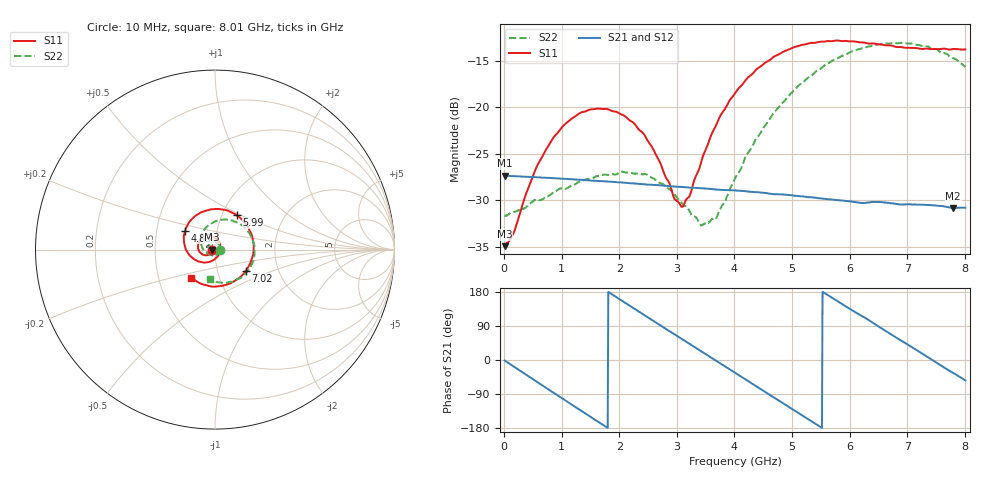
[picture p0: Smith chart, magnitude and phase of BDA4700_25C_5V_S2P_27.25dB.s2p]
!Agilent Technologies,E5071B,MY42404982,A.09.10
!Date: Mon Oct 20 13:40:14 2025
!Data & Calibration Information:
!Freq	S11:SOLT2(ON)	S21:SOLT2(ON)	S12:SOLT2(ON)	S22:SOLT2(ON)
# Hz S RI R 50
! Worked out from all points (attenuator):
!   801 points, 10 MHz to 8.01 GHz, reference 50 ohm
!   highest |S21| = -27.32 dB at 10 MHz (marker M1); lowest = -30.8 dB at 7.8 GHz (marker M2)
!   lowest |S11| = -34.9 dB at 10 MHz (marker M3), VSWR 1.04, Z = 48.2 - j0.0925 ohm
!   |S11| at or under -10 dB: start of sweep to end of sweep
!   |S22| runs from -32.7 to -13.0 dB; largest |S21 - S12| = 0.00037
!   S11 on the Smith chart (normalised r, x): 10 MHz: 0.96, -0.00; 4.83 GHz: 0.70, +0.15; 5.99 GHz: 1.17, +0.47; 7.02 GHz: 1.37, -0.34; 8.01 GHz: 0.73, -0.24
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1e7  -0.0179 -0.000958  0.043 -0.000934  0.0431 -0.00095  0.0261 -0.000852
1.6e8  -0.0187 -0.00943  0.041 -0.0121  0.041 -0.0121  0.0263 -0.0075
5.3e8  -0.0349 -0.0284  0.0251 -0.0339  0.025 -0.0339  0.0161 -0.0275
7.7e8  -0.0537 -0.0315  0.00913 -0.0408  0.00905 -0.0408  0.00105 -0.0335
1.35e9  -0.094 0.00478  -0.0288 -0.0289  -0.0288 -0.0289  -0.036 -0.0178
2.09e9  -0.0515 0.0738  -0.0348 0.0183  -0.0349 0.0184  -0.0293 0.0339
2.42e9  -0.00922 0.0718  -0.0193 0.0335  -0.0193 0.0335  -0.00496 0.0434
2.68e9  0.0178 0.0494  -0.00321 0.0381  -0.0032 0.0381  0.0128 0.0375
2.96e9  0.0299 0.0119  0.0142 0.0347  0.0142 0.0347  0.0255 0.0226
3.11e9  0.0276 -0.0103  0.0223 0.0299  0.0223 0.0299  0.028 0.0107
3.42e9  0.00124 -0.0505  0.0338 0.0146  0.0338 0.0146  0.0196 -0.0124
3.54e9  -0.015 -0.0615  0.0358 0.00747  0.0358 0.00739  0.013 -0.0203
3.7e9  -0.043 -0.0703  0.0361 -0.00222  0.0361 -0.00238  -0.000734 -0.0261
4.01e9  -0.1016 -0.0616  0.0298 -0.0198  0.0299 -0.0197  -0.0323 -0.0258
4.83e9  -0.1671 0.1055  -0.0131 -0.0314  -0.013 -0.0314  -0.0771 0.072
5.35e9  -0.0709 0.2103  -0.0313 -0.00966  -0.0314 -0.00974  -0.0152 0.1479
5.99e9  0.1212 0.191  -0.0226 0.0216  -0.0227 0.0216  0.1289 0.1482
6.68e9  0.2149 -0.00914  0.00988 0.029  0.00996 0.0291  0.22 1.24e-05
7.02e9  0.1728 -0.1173  0.0232 0.0192  0.0233 0.0192  0.2002 -0.0909
7.43e9  0.0572 -0.1975  0.0298 0.000274  0.0299 0.000214  0.1198 -0.1671
7.8e9  -0.0706 -0.1933  0.0237 -0.0162  0.0238 -0.0163  0.0203 -0.1827
8.01e9  -0.1317 -0.1569  0.017 -0.0233  0.017 -0.0234  -0.0304 -0.1621
